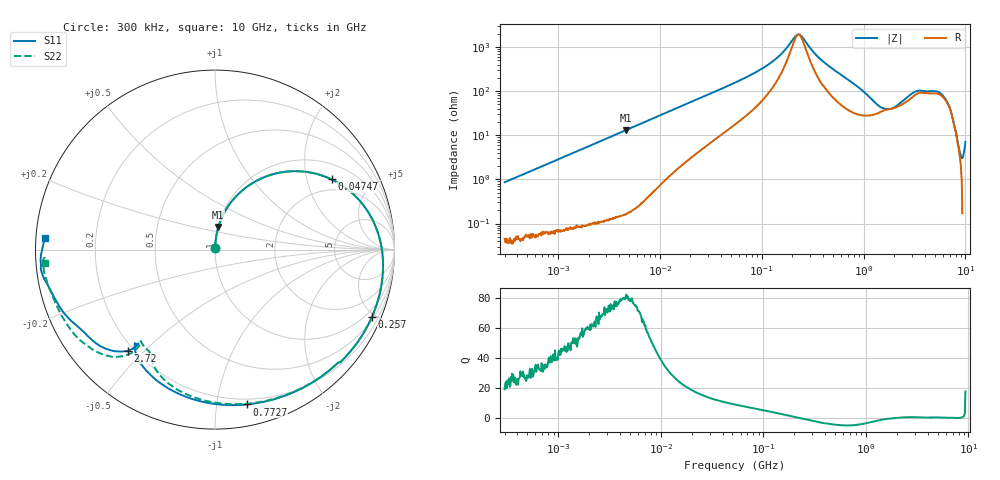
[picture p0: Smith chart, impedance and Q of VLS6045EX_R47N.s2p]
! S-Parameter Data Generated by TDK Corporation
! Copyright(C) 2019 TDK Corporation.
! All Rights Reserved.
! TDK P/N: VLS6045EX-R47N (Inductor)
! Property: L=470nH at 100kHz
! Size(LxWxT): 6x6x4.5mm
! Model Type: s2p (Touchstone File Format Version 1.0)
! Frequency: DC=Yes Start=0.3MHz Stop=10000MHz 802points Log-sweep
! Model Generated on May 10, 2019
! Port Assignments:
!  1 ---@@@--- 2
! Applicable Conditions:
!  Temperature = 25 degC
!  DC Bias Current = 0 A
!  Small Signal Operation
! Terms and conditions regarding TDK Simulation Models
! (1)This simulation model is being provided solely for informational purposes. Please refer to the specifications of the products in terms of detailed characteristics of such products.
! (2)In no event shall TDK Corporation of any of its subsidiaries be liable for any loss or damage arising, directly or indirectly,
!  From any information contained in this simulation model, including, but not limited to loss or damages arising from any inaccuracies, omissions or errors in connection with such information.
! (3)Any and all copyrights on this simulation model are owned by TDK Corporation.
!  Duplication or redistribution of this simulation model without prior written permission from TDK Corporation is prohibited.
! (4)This simulation model is subject to any modification or change without any prior notice.
! (5)Neither TDK Corporation nor any of its subsidiaries shall make any warranty, express or implied,
!  Including but not limited to the correctness, implied warranties of merchantability and fitness for a particular purpose with respect to this simulation models.
! (6)The use of this simulation model shall be deemed to have consented to the terms and conditions hereof.
# Hz S MA R 50
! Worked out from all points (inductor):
!   801 points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, 300 kHz to 10 GHz, reference 50 ohm
!   read as one part in series: L = 455 nH near 318.3 kHz
!   highest Q = 79.3 at 4.673 MHz (marker M1), where L = 447 nH
!   self-resonance near 230.5 MHz
!   S11 on the Smith chart (normalised r, x): 300 kHz: 1.00, +0.02; 47.47 MHz: 1.54, +2.83; 257 MHz: 0.60, -4.76; 772.7 MHz: 0.16, -1.21; 2.72 GHz: 0.18, -0.45; 10 GHz: 0.02, +0.03
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300000  0.008467 86.3  0.9995 -0.5  0.9995 -0.5  0.008472 86.6
1713600  0.04693 86.2  0.998 -2.8  0.9982 -2.8  0.04692 86.1
4673027  0.1268 81.6  0.9903 -7.7  0.9903 -7.7  0.1268 81.6
9671944  0.2559 72.9  0.9603 -15.6  0.9603 -15.6  0.2558 72.9
2.53611e7  0.5537 50.5  0.7966 -35.7  0.7966 -35.7  0.5536 50.5
4.746882e7  0.758 31.1  0.5781 -52.9  0.578 -52.9  0.7579 31.1
5.477226e7  0.7955 26.6  0.5212 -56.8  0.5212 -56.8  0.7955 26.6
1.258969e8  0.9279 0.8  0.205 -74.4  0.205 -74.4  0.9279 0.9
2.22675e8  0.9513 -18.0  0.04911 -30.2  0.04913 -30.3  0.9511 -17.9
2.569609e8  0.9513 -23.4  0.05827 12.5  0.05827 12.4  0.951 -23.3
3.126428e8  0.9483 -31.3  0.1048 32.5  0.1048 32.4  0.948 -31.2
4.627802e8  0.9235 -49.3  0.2113 27.9  0.2112 27.9  0.9226 -49.3
7.726947e8  0.8806 -78.4  0.3334 2.1  0.3333 2.1  0.8753 -79.0
1.260284e9  0.8142 -109.2  0.396 -35.1  0.396 -35.1  0.7771 -111.5
1.767019e9  0.7274 -127.4  0.376 -69.1  0.3762 -69.3  0.6737 -124.2
2.142542e9  0.6771 -129.4  0.3393 -95.9  0.3386 -96.0  0.6574 -129.0
2.720446e9  0.7427 -130.7  0.2134 -130.9  0.2128 -130.9  0.756 -129.5
3.472057e9  0.8436 -141.7  0.1065 -142.8  0.1065 -142.8  0.8591 -137.4
4.632637e9  0.8855 -152.3  0.06641 -153.0  0.06618 -152.9  0.9049 -146.0
6.899057e9  0.9523 -168.0  0.027 -154.5  0.02723 -154.2  0.9462 -166.4
8.322921e9  0.9739 -176.0  0.0231 -143.0  0.02341 -143.5  0.9607 -175.1
1e10  0.9515 176.1  0.02678 -135.6  0.02678 -136.2  0.9497 -175.5
